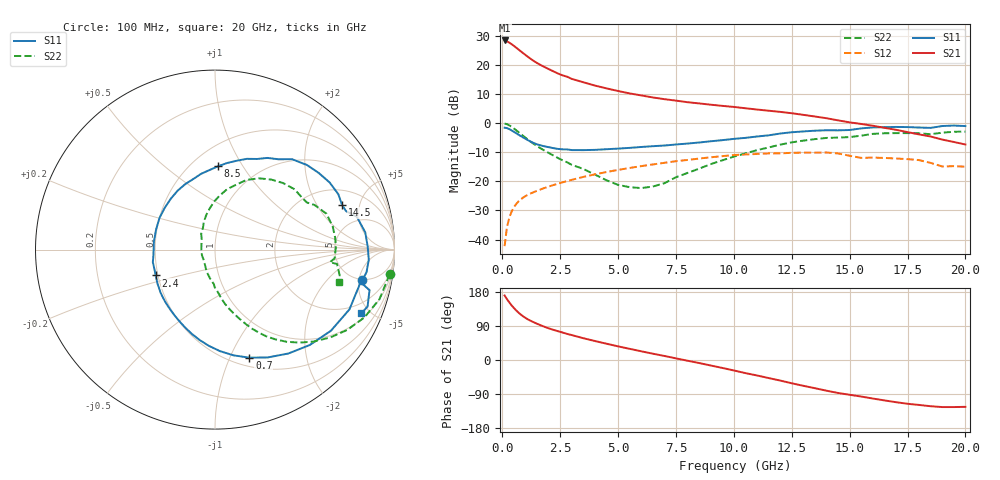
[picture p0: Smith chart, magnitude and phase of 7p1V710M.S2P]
! Infineon Technologies  Discrete & RF Semiconductors
! bfp620
! VCE =  1.7 V,  IC =  10 mA
! Common Emitter S-Parameters:  Sep 2002
# GHz  S  MA  R  50
!  f  S11  S21  S12  S22
! GHz  MAG  ANG  MAG  ANG  MAG  ANG  MAG  ANG
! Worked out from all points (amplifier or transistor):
!   59 points, 100 MHz to 20 GHz, reference 50 ohm
!   highest |S21| = 28.4 dB at 100 MHz (marker M1)
!   |S21| within 3 dB of that: start of sweep to 684.4 MHz
!   unconditionally stable (mu >= 1): 4.083 GHz to 10.61 GHz; 17.12 GHz to end of sweep
!   at 1 GHz: K = 0.49, MSG = 24.2 dB, |S12| = -25.1 dB
!   at 5.5 GHz: K = 1.04, MAG = 11.5 dB, |S12| = -15.4 dB
!   at 20 GHz: K = 1.34, MAG = 0.3 dB, |S12| = -15.0 dB
!   S11 on the Smith chart (normalised r, x): 100 MHz: 4.94, -5.45; 700 MHz: 0.59, -1.19; 2.4 GHz: 0.49, -0.16; 8.5 GHz: 0.66, +0.78; 14.5 GHz: 2.96, +3.38; 20 GHz: 1.31, -4.42
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0.1  0.8342 -11.6  26.23 170.3  0.0077 82.2  0.983 -8.1
0.2  0.8197 -24.0  25.35 160.7  0.0162 77.6  0.9569 -16.8
0.3  0.7884 -35.0  24.09 152.2  0.0236 72.6  0.9143 -24.4
0.4  0.7493 -45.2  22.66 144.4  0.0301 68.2  0.8626 -31.2
0.5  0.7085 -54.8  21.18 137.3  0.0358 64.3  0.8075 -37.3
0.7  0.6321 -72.3  18.36 125.0  0.0452 58.2  0.6995 -47.8
0.8  0.598 -80.1  17.08 119.8  0.0491 55.8  0.6498 -52.2
1  0.5371 -93.7  14.79 111.1  0.0557 52.1  0.5613 -59.4
1.3  0.4655 -110.8  12.09 101.2  0.0638 48.5  0.4562 -67.0
1.5  0.4325 -120.8  10.76 95.7  0.0688 46.9  0.4028 -71.0
1.8  0.4011 -134.0  9.273 88.2  0.0763 45.1  0.3413 -76.3
2.4  0.3604 -156.5  7.11 76.1  0.091 41.9  0.252 -84.6
3  0.344 -175.2  5.738 65.8  0.106 38.4  0.1919 -92.0
3.5  0.3434 172.5  5.025 57.5  0.1191 35.3  0.1632 -99.7
5  0.3644 140.1  3.555 36.0  0.1572 24.3  0.0869 -135.2
7  0.4118 106.9  2.575 10.7  0.2079 7.8  0.0928 142.9
8.5  0.4642 88.0  2.176 -8.0  0.2459 -6.5  0.1649 112.3
10.5  0.5571 65.0  1.797 -34.6  0.2896 -29.0  0.3017 85.1
13.5  0.7403 30.3  1.297 -74.4  0.3108 -62.7  0.5302 44.4
14.5  0.7505 19.4  1.114 -87.0  0.3015 -77.6  0.5637 31.3
17  0.8586 -3.7  0.768 -111.3  0.2465 -93.9  0.6732 5.4
20  0.8882 -23.6  0.429 -123.6  0.1785 -105.4  0.7145 -14.8
